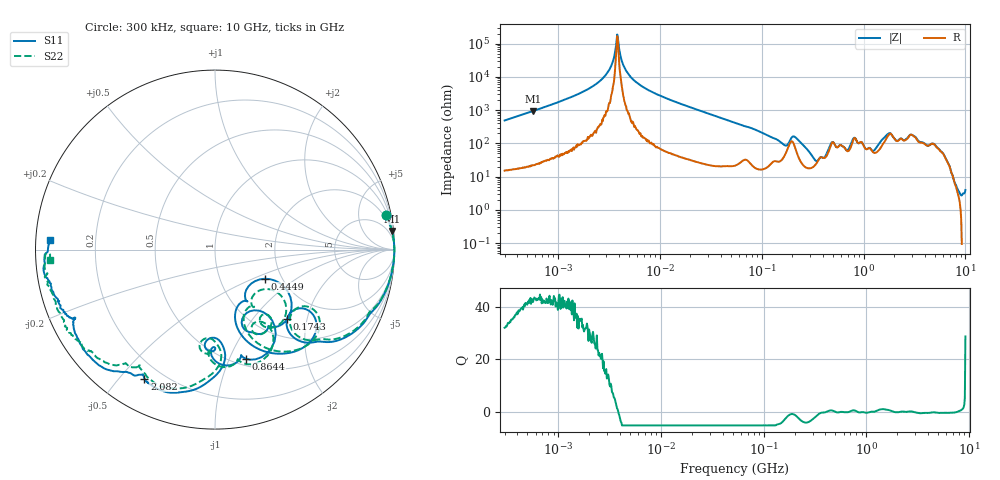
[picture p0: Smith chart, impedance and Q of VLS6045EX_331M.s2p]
! S-Parameter Data Generated by TDK Corporation
! Copyright(C) 2019 TDK Corporation.
! All Rights Reserved.
! TDK P/N: VLS6045EX-331M (Inductor)
! Property: L=330uH at 100kHz
! Size(LxWxT): 6x6x4.5mm
! Model Type: s2p (Touchstone File Format Version 1.0)
! Frequency: DC=Yes Start=0.3MHz Stop=10000MHz 802points Log-sweep
! Model Generated on May 10, 2019
! Port Assignments:
!  1 ---@@@--- 2
! Applicable Conditions:
!  Temperature = 25 degC
!  DC Bias Current = 0 A
!  Small Signal Operation
! Terms and conditions regarding TDK Simulation Models
! (1)This simulation model is being provided solely for informational purposes. Please refer to the specifications of the products in terms of detailed characteristics of such products.
! (2)In no event shall TDK Corporation of any of its subsidiaries be liable for any loss or damage arising, directly or indirectly,
!  From any information contained in this simulation model, including, but not limited to loss or damages arising from any inaccuracies, omissions or errors in connection with such information.
! (3)Any and all copyrights on this simulation model are owned by TDK Corporation.
!  Duplication or redistribution of this simulation model without prior written permission from TDK Corporation is prohibited.
! (4)This simulation model is subject to any modification or change without any prior notice.
! (5)Neither TDK Corporation nor any of its subsidiaries shall make any warranty, express or implied,
!  Including but not limited to the correctness, implied warranties of merchantability and fitness for a particular purpose with respect to this simulation models.
! (6)The use of this simulation model shall be deemed to have consented to the terms and conditions hereof.
# Hz S MA R 50
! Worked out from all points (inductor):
!   801 points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, 300 kHz to 10 GHz, reference 50 ohm
!   read as one part in series: L = 257 uH near 318.3 kHz
!   highest Q = 42.8 at 567.7 kHz (marker M1), where L = 262 uH
!   self-resonance near 3.822 MHz
!   S11 on the Smith chart (normalised r, x): 300 kHz: 1, +10; 174.3 MHz: 1.36, -1.52; 444.9 MHz: 1.64, -0.59; 864.4 MHz: 0.57, -1.16; 2.082 GHz: 0.13, -0.58; 10 GHz: 0.04, +0.03
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300000  0.9732 11.3  0.1992 -76.9  0.1994 -76.9  0.9731 11.3
567737  0.9914 6.0  0.106 -82.7  0.106 -82.7  0.9913 6.0
1713600  0.9987 1.5  0.02927 -86.7  0.02932 -86.9  0.9987 1.5
3016998  0.9994 0.2  0.007979 -85.7  0.008006 -85.8  0.9994 0.2
3419615  0.9994 -0.1  0.003858 -81.9  0.003886 -81.7  0.9994 -0.1
3822232  0.9995 -0.3  0.0005329 -26.9  0.0005491 -17.1  0.9995 -0.3
5044683  0.9993 -1.0  0.009076 85.5  0.009114 85.3  0.9994 -0.9
9671944  0.9984 -2.9  0.03482 85.7  0.03482 85.7  0.9986 -2.8
5.477226e7  0.962 -18.1  0.2296 69.1  0.2297 69.1  0.961 -17.7
1.177683e8  0.8274 -38.4  0.4697 45.3  0.4696 45.3  0.8288 -37.1
1.743231e8  0.5564 -43.8  0.571 12.8  0.571 12.8  0.5626 -41.8
2.102074e8  0.7276 -39.9  0.4132 21.9  0.4132 21.9  0.733 -37.8
3.126428e8  0.4806 -73.4  0.7378 1.8  0.7378 1.8  0.4978 -68.5
4.448526e8  0.3217 -30.3  0.6447 -37.8  0.6447 -37.8  0.3713 -36.4
5.046115e8  0.5578 -43.1  0.4407 -33.7  0.4407 -33.7  0.5499 -50.0
7.318083e8  0.4183 -54.4  0.5347 -57.7  0.5348 -57.7  0.4836 -56.7
8.643532e8  0.633 -74.1  0.3644 -48.7  0.3645 -48.7  0.6509 -76.2
1.323741e9  0.4955 -88.9  0.4756 -87.7  0.4761 -87.7  0.4962 -92.6
1.767019e9  0.8225 -104.5  0.1551 -115.3  0.1557 -115.4  0.809 -107.3
2.08171e9  0.8196 -118.7  0.1671 -99.5  0.1677 -99.8  0.7737 -123.3
3.093017e9  0.9171 -138.1  0.07343 -112.2  0.07295 -112.7  0.8834 -135.6
1e10  0.9191 176.6  0.05518 -150.5  0.05506 -150.4  0.9238 -176.3
